(* Logix 5000 AddOnInstructionDefinition export Banner_IOLM_Param_C_v4; software revision 33.03 *)

TYPE Banner_IOL_Port_v4 :   // UDT that has all of the data items necessary to communicate with a specific Port on a IO-Link Master
STRUCT
   Port_Controlled : INT;   // Each bit represents a port on an IO-Link Master. Set to 1 to tell AOI to control that port.
   Port_Activate : INT;   // Each bit represents a port on an IO-Link Master. When ON that port will process any commands in queue.
   Port_Read : INT;   // Each bit represents a port on an IO-Link Master. Used to determine when device AOI has requested a Read command.
   Port_Write : INT;   // Each bit represents a port on an IO-Link Master. Used to determine when device AOI has requested a Write command.
   Port_RW_Complete : INT;   // Each bit represents a port on an IO-Link Master. Tells device AOI that Read or Write request has been completed.
   Port_Device_Read : INT;
   Data_Transfer : SINT[190];   // Array to transfer data from IO-Master to device AOIs.
END_STRUCT
END_TYPE

TYPE Banner_IOLM_EL_v4 :   // Error Log for Messages to IOLM.
STRUCT
   RW : SINT;   // 0 = Read, 1 = Write, 3 = AOI Failure.
   Port : SINT;   // Port number that generated error.
   Index : INT;   // IO-Link Index for generated error.
END_STRUCT
END_TYPE

TYPE Banner_IOLMC_v4 :   // UDT to control IO-Link Masters. Modified for Comtrol Masters.
STRUCT
   Message_Source_Data : SINT[380];   // Array used to generate the source data for an Explicit Message
   Message_Destination_Data : SINT[380];   // Array that stores the data from the IO-Link sensor for an Explicit Message.
   Error_Log : Banner_IOLM_EL_v4[10];
   Error_Write_Retry : BOOL;
   Num_Error_MSGS : DINT;   // 0 = While waiting for a command, 1 = Processing command
   IO_Link_Master_Busy : BOOL;
   AOI_Reset : BOOL;   // Resets AOI.
   Port_Data : Banner_IOL_Port_v4;
   Halt_Operation : BOOL;
   AOI_Halted : BOOL;
END_STRUCT
END_TYPE

ADD_ON_INSTRUCTION Banner_IOLM_Param_C_v4   (* revision 4.4, vendor Banner Engineering *)
// AOI that controls a Comtrol IO-Link Master with Banner devices for parameter data operations.
// Revision note:
// Fixed an issue with Halt AOI causing a Major fault due to array going out of index.
VAR_IN_OUT
   Message : MESSAGE; {required}   // Message used to gather data from a device plugged into an Allen Bradley IO-Link Master.
   IOLM : Banner_IOLMC_v4; {required}
END_VAR
VAR
   Lock : DINT; {access None}
   Disable_Timer : BOOL; {access None}
   Byte_Length : SINT; {access None}
   Current_Port : INT; {access None}   // Current port to communicate with via the IO-Link Master.
   Array_Index : DINT; {access None}
   Data_Index : DINT; {access None}
   Message_Timer : TIMER := (PRE := 100); {access None}
   Message_Timer2 : TIMER := (PRE := 5000); {access None}
   Error_Index : DINT; {access None}
   Temp_Index : INT; {access None}
END_VAR

ROUTINE Logic   (* ladder *)
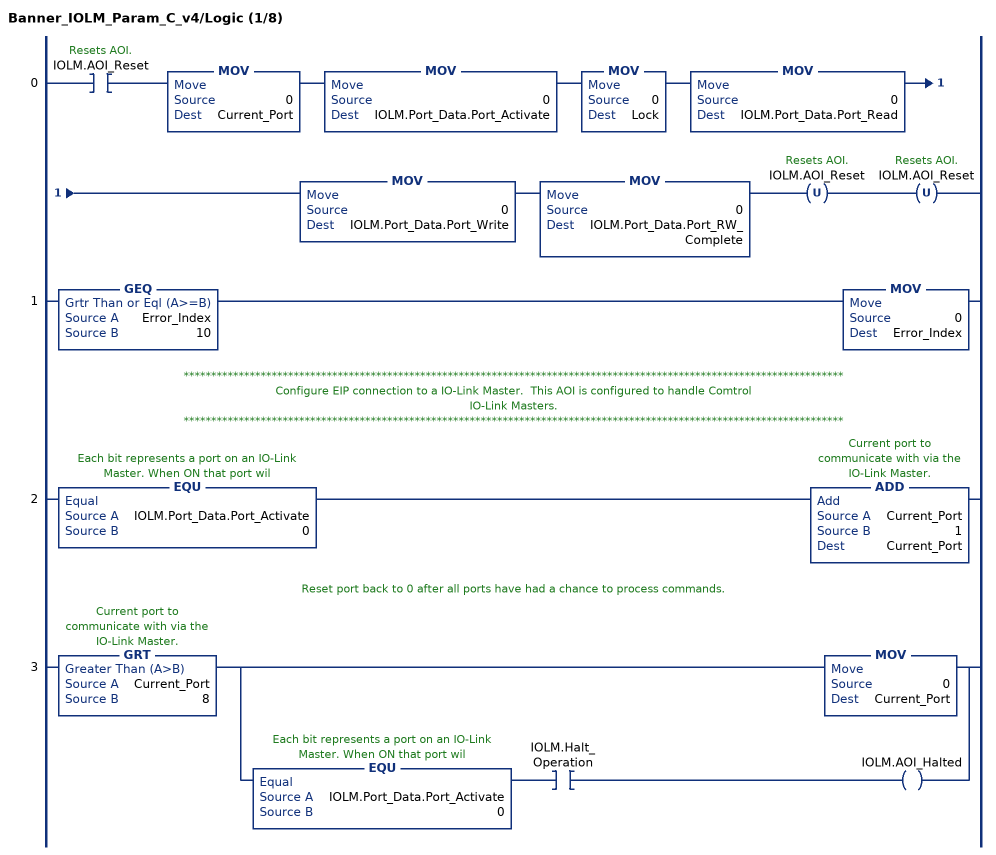
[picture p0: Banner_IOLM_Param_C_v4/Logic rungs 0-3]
   0: XIC(IOLM.AOI_Reset)MOV(0,Current_Port)MOV(0,IOLM.Port_Data.Port_Activate)MOV(0,Lock)MOV(0,IOLM.Port_Data.Port_Read)MOV(0,IOLM.Port_Data.Port_Write)MOV(0,IOLM.Port_Data.Port_RW_Complete)OTU(IOLM.AOI_Reset)OTU(IOLM.AOI_Reset);
   1: GEQ(Error_Index,10)MOV(0,Error_Index);
   // ************************************************************************************************************************
   // Configure EIP connection to a IO-Link Master.  This AOI is configured to handle Comtrol
   // IO-Link Masters.
   // ************************************************************************************************************************
   2: EQU(IOLM.Port_Data.Port_Activate,0)ADD(Current_Port,1,Current_Port);
   // Reset port back to 0 after all ports have had a chance to process commands.
   3: GRT(Current_Port,8)[MOV(0,Current_Port) ,EQU(IOLM.Port_Data.Port_Activate,0) XIC(IOLM.Halt_Operation) OTE(IOLM.AOI_Halted) ];
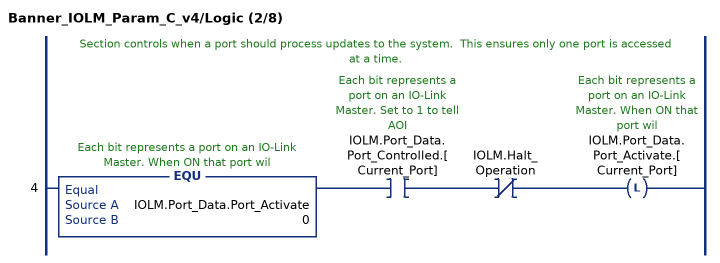
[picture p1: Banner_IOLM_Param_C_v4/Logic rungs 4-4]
   // Section controls when a port should process updates to the system.  This ensures only one port is accessed at a time.
   4: EQU(IOLM.Port_Data.Port_Activate,0)XIC(IOLM.Port_Data.Port_Controlled.[Current_Port])XIO(IOLM.Halt_Operation)OTL(IOLM.Port_Data.Port_Activate.[Current_Port]);
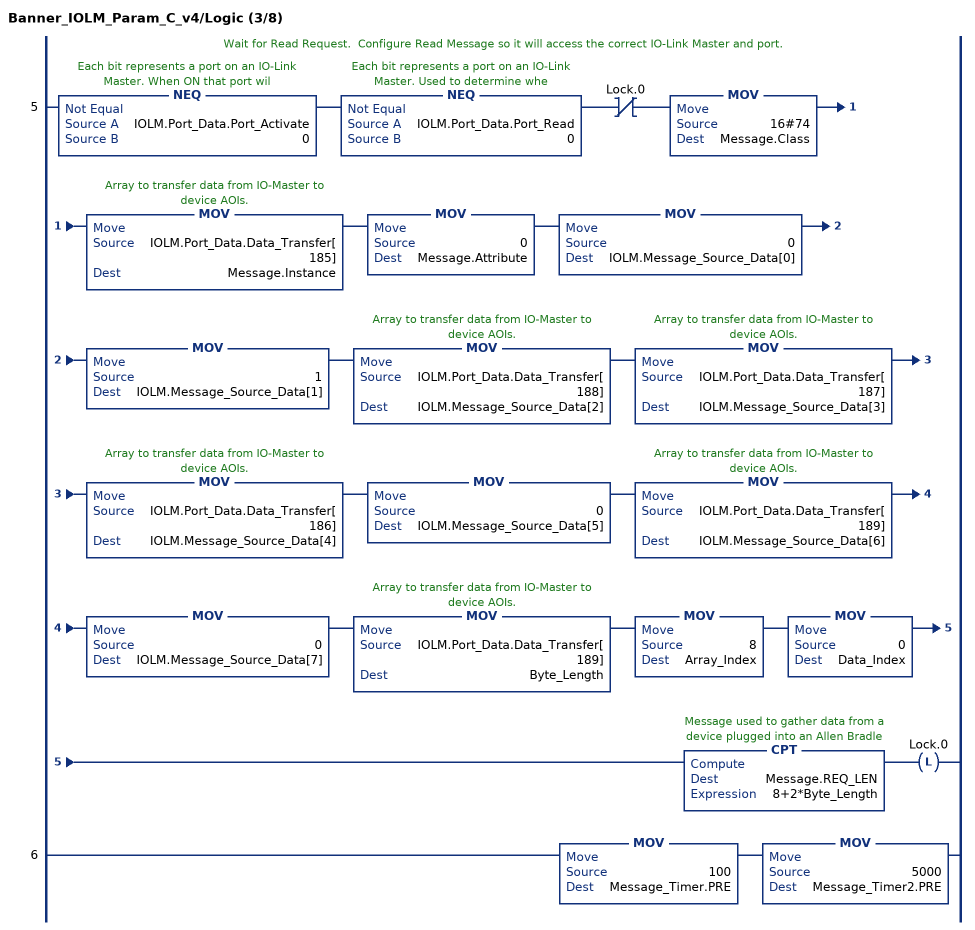
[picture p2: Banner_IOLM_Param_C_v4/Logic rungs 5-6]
   // Wait for Read Request.  Configure Read Message so it will access the correct IO-Link Master and port.
   5: NEQ(IOLM.Port_Data.Port_Activate,0)NEQ(IOLM.Port_Data.Port_Read,0)XIO(Lock.0)MOV(16#74,Message.Class)MOV(IOLM.Port_Data.Data_Transfer[185],Message.Instance)MOV(0,Message.Attribute)MOV(0,IOLM.Message_Source_Data[0])MOV(1,IOLM.Message_Source_Data[1])MOV(IOLM.Port_Data.Data_Transfer[188],IOLM.Message_Source_Data[2])MOV(IOLM.Port_Data.Data_Transfer[187],IOLM.Message_Source_Data[3])MOV(IOLM.Port_Data.Data_Transfer[186],IOLM.Message_Source_Data[4])MOV(0,IOLM.Message_Source_Data[5])MOV(IOLM.Port_Data.Data_Transfer[189],IOLM.Message_Source_Data[6])MOV(0,IOLM.Message_Source_Data[7])MOV(IOLM.Port_Data.Data_Transfer[189],Byte_Length)MOV(8,Array_Index)MOV(0,Data_Index)CPT(Message.REQ_LEN,8+2*Byte_Length)OTL(Lock.0);
   6: MOV(100,Message_Timer.PRE)MOV(5000,Message_Timer2.PRE);
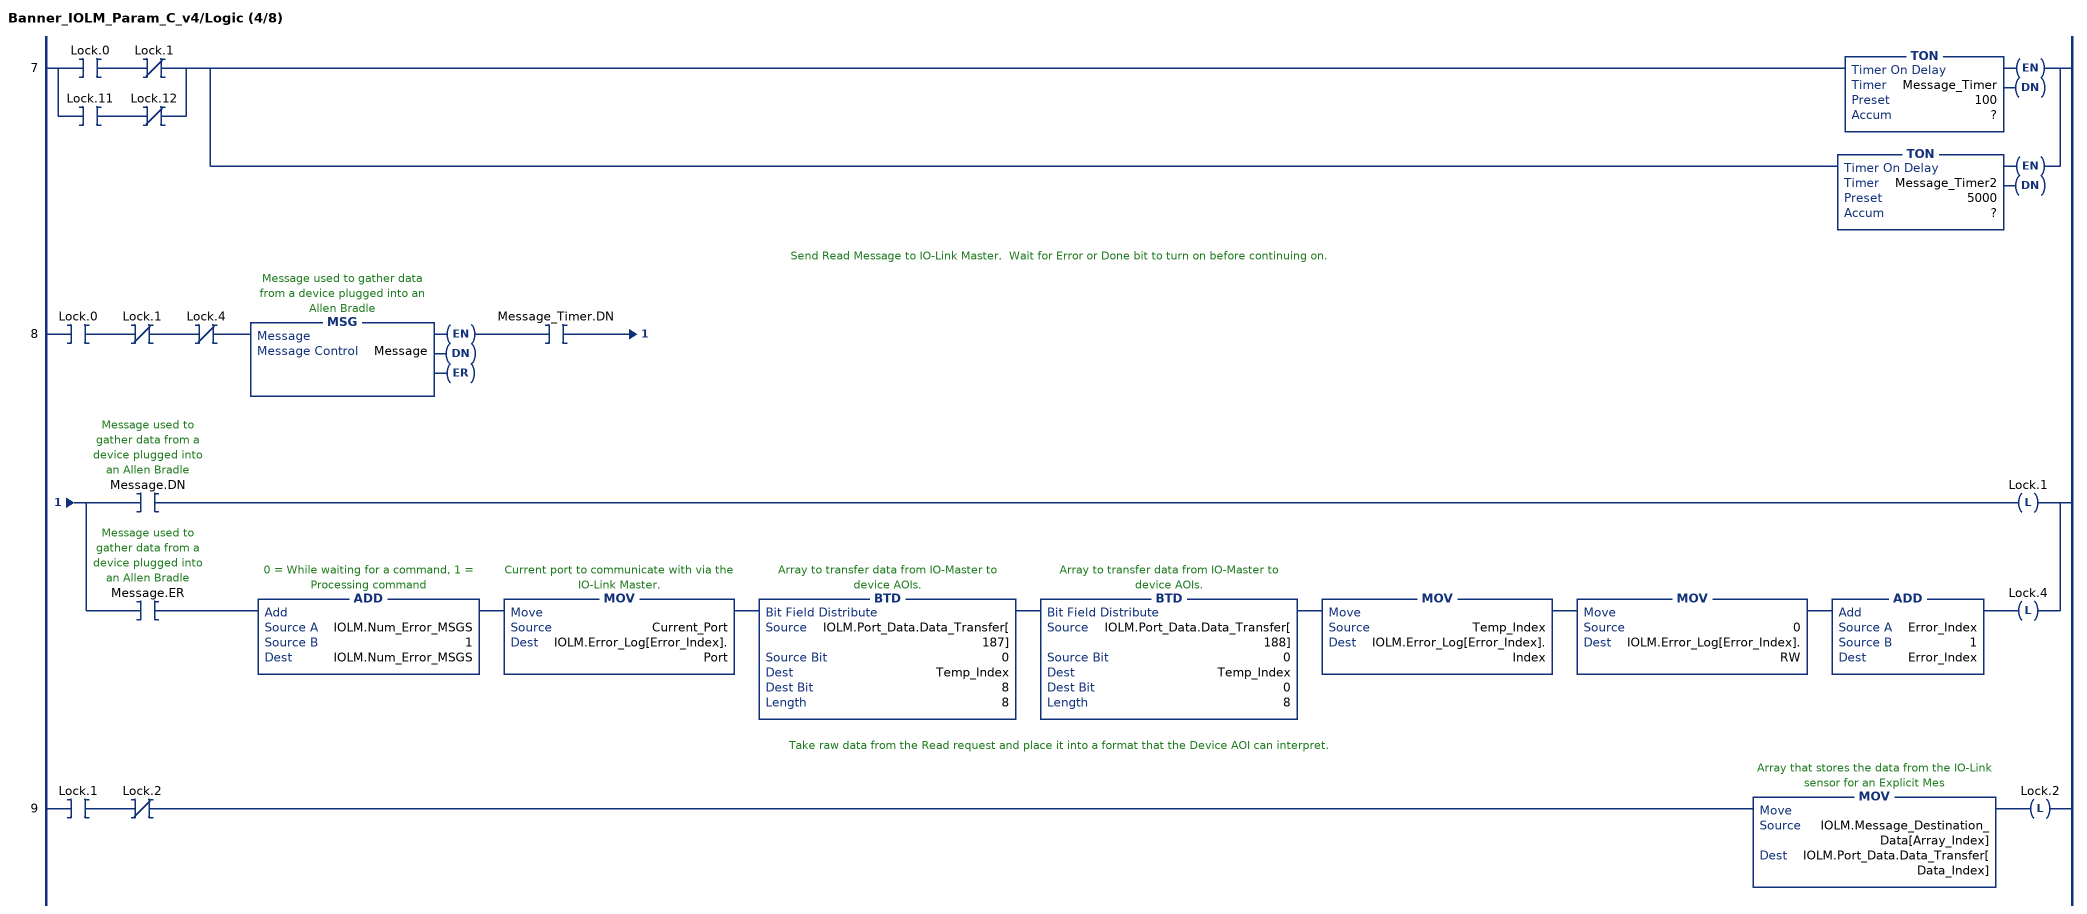
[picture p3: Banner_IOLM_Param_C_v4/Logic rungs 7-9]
   7: [XIC(Lock.0) XIO(Lock.1) ,XIC(Lock.11) XIO(Lock.12) ][TON(Message_Timer,?,?) ,TON(Message_Timer2,?,?) ];
   // Send Read Message to IO-Link Master.  Wait for Error or Done bit to turn on before continuing on.
   8: XIC(Lock.0)XIO(Lock.1)XIO(Lock.4)MSG(Message)XIC(Message_Timer.DN)[XIC(Message.DN) OTL(Lock.1) ,XIC(Message.ER) ADD(IOLM.Num_Error_MSGS,1,IOLM.Num_Error_MSGS) MOV(Current_Port,IOLM.Error_Log[Error_Index].Port) BTD(IOLM.Port_Data.Data_Transfer[187],0,Temp_Index,8,8) BTD(IOLM.Port_Data.Data_Transfer[188],0,Temp_Index,0,8) MOV(Temp_Index,IOLM.Error_Log[Error_Index].Index) MOV(0,IOLM.Error_Log[Error_Index].RW) ADD(Error_Index,1,Error_Index) OTL(Lock.4) ];
   // Take raw data from the Read request and place it into a format that the Device AOI can interpret.
   9: XIC(Lock.1)XIO(Lock.2)MOV(IOLM.Message_Destination_Data[Array_Index],IOLM.Port_Data.Data_Transfer[Data_Index])OTL(Lock.2);
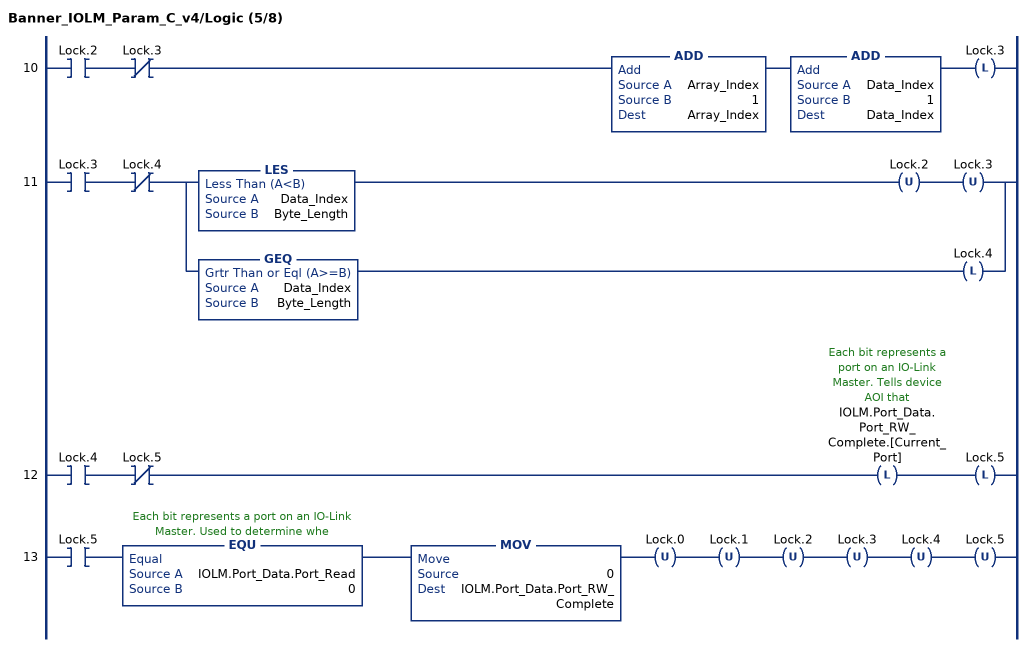
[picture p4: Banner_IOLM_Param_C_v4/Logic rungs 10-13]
   10: XIC(Lock.2)XIO(Lock.3)ADD(Array_Index,1,Array_Index)ADD(Data_Index,1,Data_Index)OTL(Lock.3);
   11: XIC(Lock.3)XIO(Lock.4)[LES(Data_Index,Byte_Length) OTU(Lock.2) OTU(Lock.3) ,GEQ(Data_Index,Byte_Length) OTL(Lock.4) ];
   12: XIC(Lock.4)XIO(Lock.5)OTL(IOLM.Port_Data.Port_RW_Complete.[Current_Port])OTL(Lock.5);
   13: XIC(Lock.5)EQU(IOLM.Port_Data.Port_Read,0)MOV(0,IOLM.Port_Data.Port_RW_Complete)OTU(Lock.0)OTU(Lock.1)OTU(Lock.2)OTU(Lock.3)OTU(Lock.4)OTU(Lock.5);
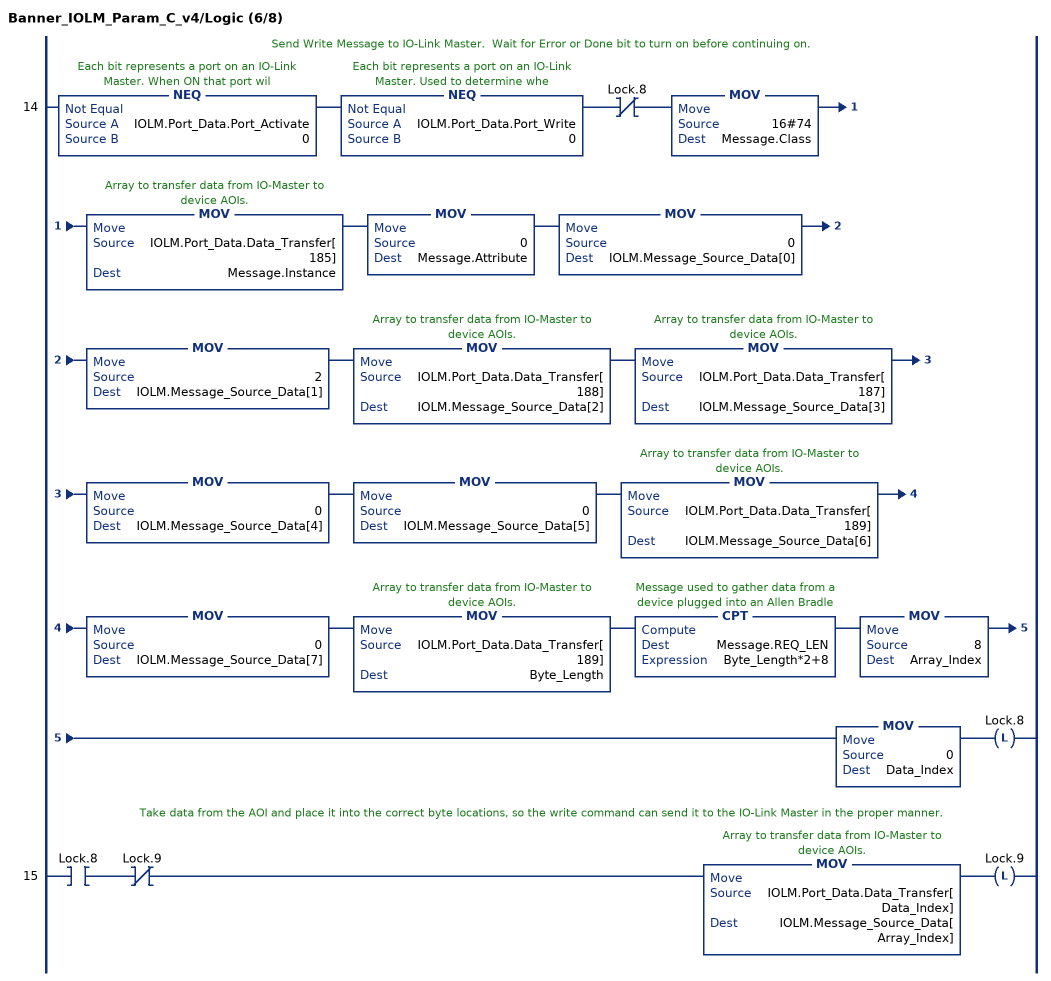
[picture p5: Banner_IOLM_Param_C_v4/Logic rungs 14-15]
   // Send Write Message to IO-Link Master.  Wait for Error or Done bit to turn on before continuing on.
   14: NEQ(IOLM.Port_Data.Port_Activate,0)NEQ(IOLM.Port_Data.Port_Write,0)XIO(Lock.8)MOV(16#74,Message.Class)MOV(IOLM.Port_Data.Data_Transfer[185],Message.Instance)MOV(0,Message.Attribute)MOV(0,IOLM.Message_Source_Data[0])MOV(2,IOLM.Message_Source_Data[1])MOV(IOLM.Port_Data.Data_Transfer[188],IOLM.Message_Source_Data[2])MOV(IOLM.Port_Data.Data_Transfer[187],IOLM.Message_Source_Data[3])MOV(0,IOLM.Message_Source_Data[4])MOV(0,IOLM.Message_Source_Data[5])MOV(IOLM.Port_Data.Data_Transfer[189],IOLM.Message_Source_Data[6])MOV(0,IOLM.Message_Source_Data[7])MOV(IOLM.Port_Data.Data_Transfer[189],Byte_Length)CPT(Message.REQ_LEN,Byte_Length*2+8)MOV(8,Array_Index)MOV(0,Data_Index)OTL(Lock.8);
   // Take data from the AOI and place it into the correct byte locations, so the write command can send it to the IO-Link Master in the proper manner.
   15: XIC(Lock.8)XIO(Lock.9)MOV(IOLM.Port_Data.Data_Transfer[Data_Index],IOLM.Message_Source_Data[Array_Index])OTL(Lock.9);
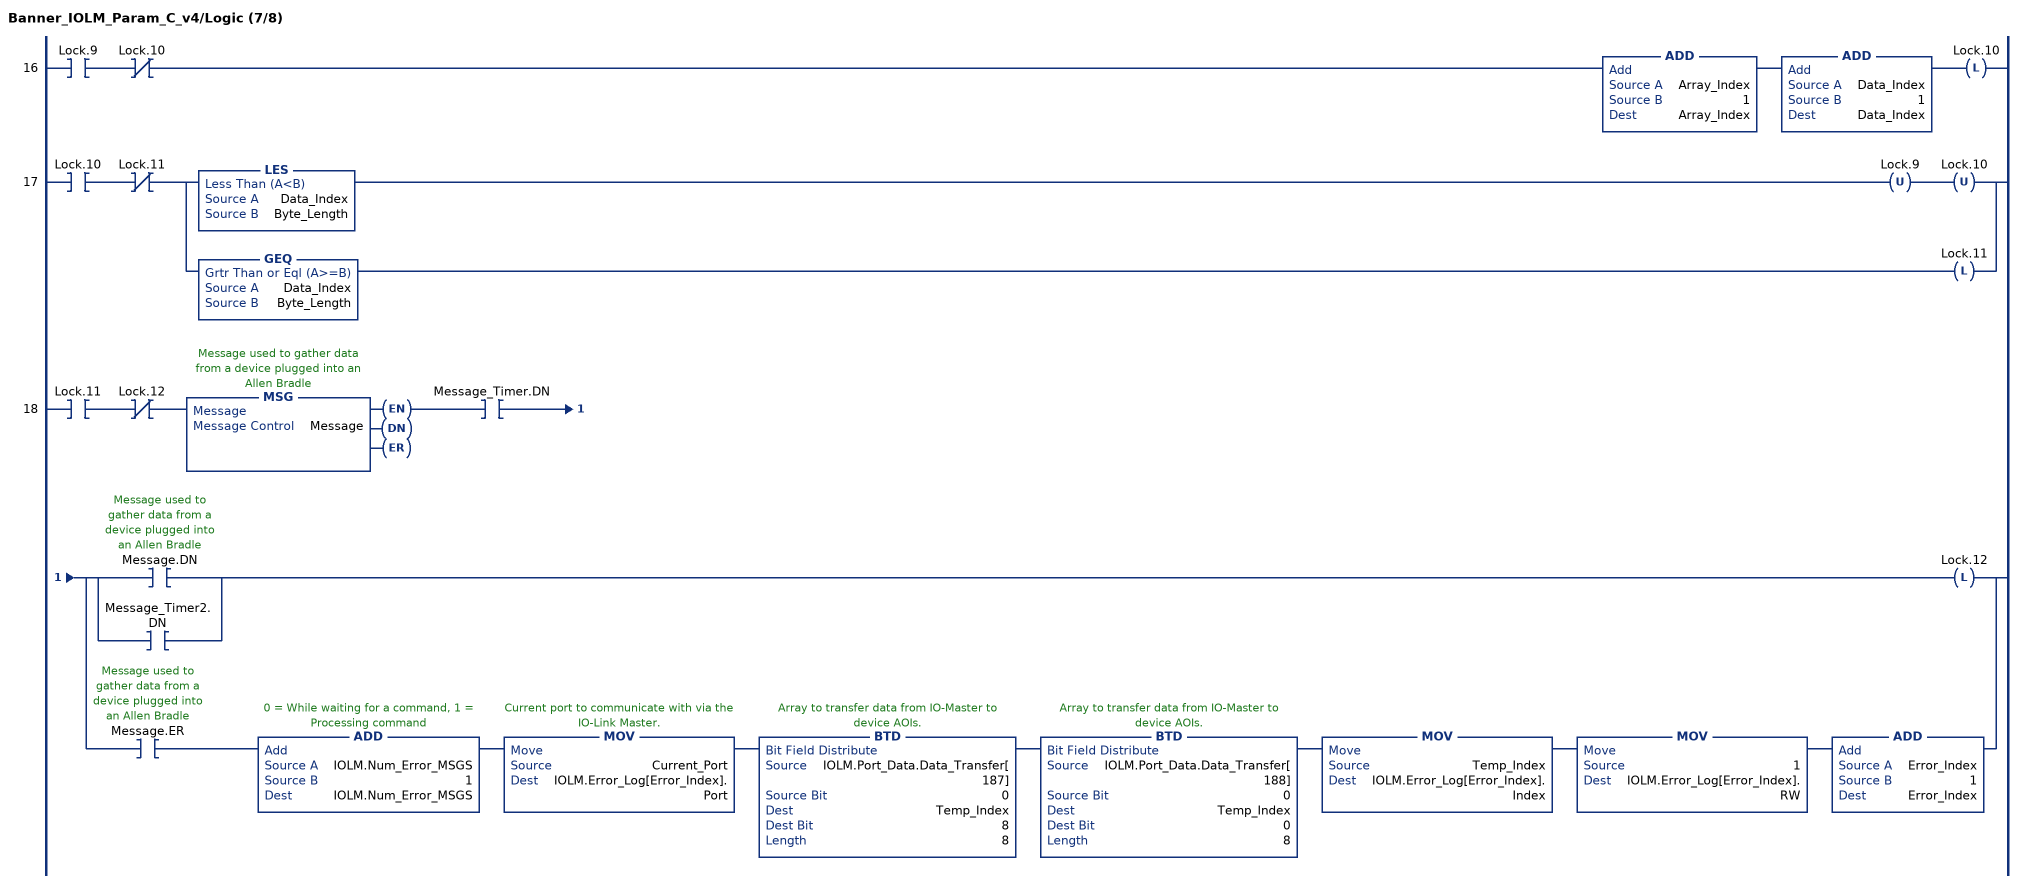
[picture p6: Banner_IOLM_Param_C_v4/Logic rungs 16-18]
   16: XIC(Lock.9)XIO(Lock.10)ADD(Array_Index,1,Array_Index)ADD(Data_Index,1,Data_Index)OTL(Lock.10);
   17: XIC(Lock.10)XIO(Lock.11)[LES(Data_Index,Byte_Length) OTU(Lock.9) OTU(Lock.10) ,GEQ(Data_Index,Byte_Length) OTL(Lock.11) ];
   18: XIC(Lock.11)XIO(Lock.12)MSG(Message)XIC(Message_Timer.DN)[[XIC(Message.DN) ,XIC(Message_Timer2.DN) ] OTL(Lock.12) ,XIC(Message.ER) ADD(IOLM.Num_Error_MSGS,1,IOLM.Num_Error_MSGS) MOV(Current_Port,IOLM.Error_Log[Error_Index].Port) BTD(IOLM.Port_Data.Data_Transfer[187],0,Temp_Index,8,8) BTD(IOLM.Port_Data.Data_Transfer[188],0,Temp_Index,0,8) MOV(Temp_Index,IOLM.Error_Log[Error_Index].Index) MOV(1,IOLM.Error_Log[Error_Index].RW) ADD(Error_Index,1,Error_Index) ];
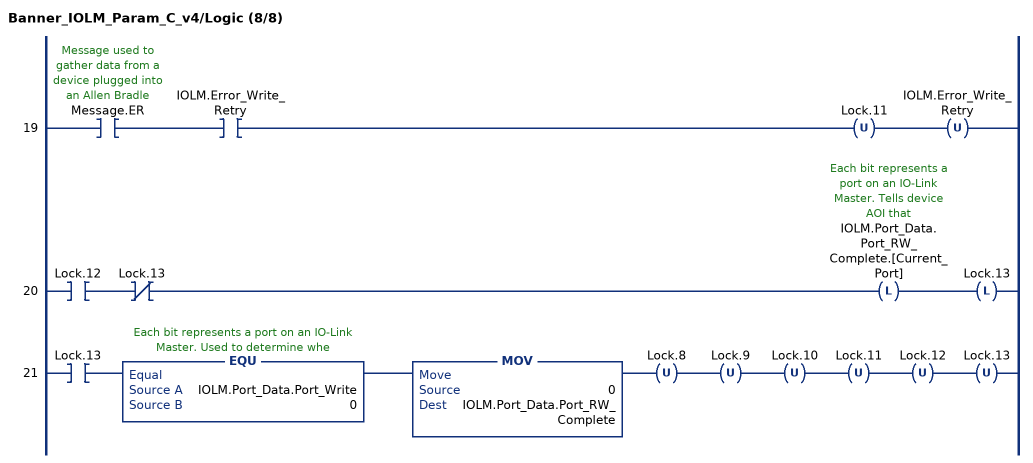
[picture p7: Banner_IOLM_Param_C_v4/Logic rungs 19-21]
   19: XIC(Message.ER)XIC(IOLM.Error_Write_Retry)OTU(Lock.11)OTU(IOLM.Error_Write_Retry);
   20: XIC(Lock.12)XIO(Lock.13)OTL(IOLM.Port_Data.Port_RW_Complete.[Current_Port])OTL(Lock.13);
   21: XIC(Lock.13)EQU(IOLM.Port_Data.Port_Write,0)MOV(0,IOLM.Port_Data.Port_RW_Complete)OTU(Lock.8)OTU(Lock.9)OTU(Lock.10)OTU(Lock.11)OTU(Lock.12)OTU(Lock.13);
END_ROUTINE
END_ADD_ON_INSTRUCTION
